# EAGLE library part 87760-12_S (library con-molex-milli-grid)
HEADER
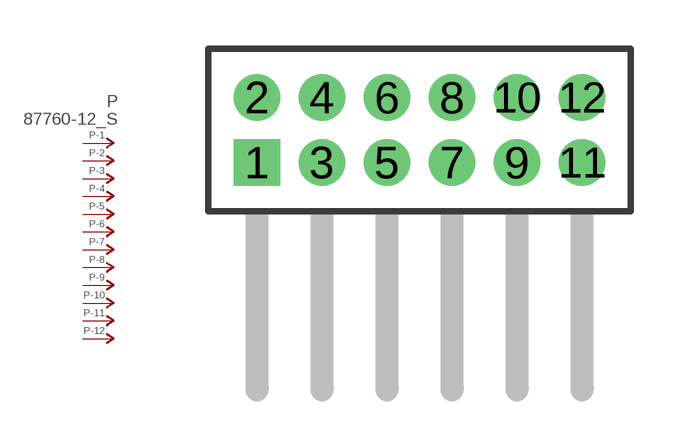
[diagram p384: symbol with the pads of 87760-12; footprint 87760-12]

Designator prefix P; gates -1=P-NV -2=P-N -3=P-N -4=P-N -5=P-N -6=P-N -7=P-N -8=P-N -9=P-N -10=P-N -11=P-N -12=P-N

## 87760-12_S  [87760-12]
1  -1:P  pas
2  -2:P  pas
3  -3:P  pas
4  -4:P  pas
5  -5:P  pas
6  -6:P  pas
7  -7:P  pas
8  -8:P  pas
9  -9:P  pas
10  -10:P  pas
11  -11:P  pas
12  -12:P  pas

## Footprint 87760-12 (pad centres in mm)
HEADER Dual Row, Right Angle
drill 0.914 square: 1 -5,-1
drill 0.914: 2 -5,1; 3 -3,-1; 4 -3,1; 5 -1,-1; 6 -1,1; 7 1,-1; 8 1,1; 9 3,-1; 10 3,1; 11 5,-1; 12 5,1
